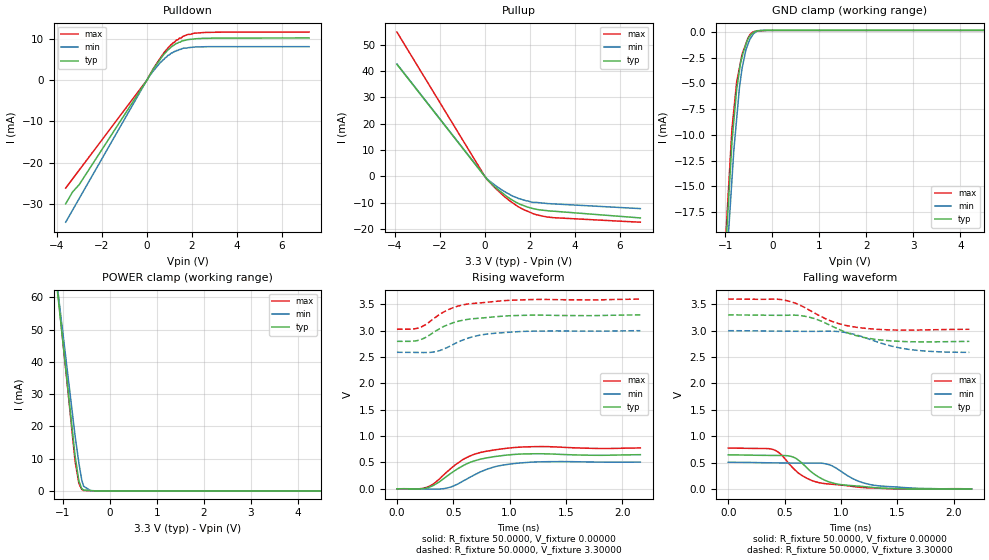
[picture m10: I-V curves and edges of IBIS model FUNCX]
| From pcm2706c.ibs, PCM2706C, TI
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[Model] FUNCX
Model_type I/O
Vinl  = 800.000mV
Vinh  = 2.00000V
Vref  = 0.00000V
Cref  = 2.00000pF
Vmeas = 1.65000V
C_comp  2.00000pF 2.00000pF 2.00000pF
| variable   typ   min   max
[Voltage Range]   3.30000V  3.00000V  3.60000V
[POWER Clamp Reference]  3.30000V  3.00000V  3.60000V
[Pullup Reference]   3.30000V  3.00000V  3.60000V
[Pulldown Reference]   0.00000V  0.00000V  0.00000V
[GND Clamp Reference]   0.00000V  0.00000V  0.00000V
[Temperature Range]   25   85   -25
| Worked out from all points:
|   slope of the pulldown table from 0 to 0.495 V, typ, clamps not added: 114 ohm
|   slope of the pullup table from 0 to 0.495 V, typ, clamps not added: 116 ohm
|   GND clamp passes 1 mA (typ) near -0.55 V on its own axis
|   POWER clamp passes 1 mA (typ) near -0.61 V on its own axis
|   rising waveform, R_fixture 50.0000, V_fixture 0.00000: 20-80 % time 296ps typ, 298ps min, 286ps max; typ from 0 V to 0.648 V
|   falling waveform, R_fixture 50.0000, V_fixture 0.00000: 20-80 % time 263ps typ, 275ps min, 265ps max; typ from 0.648 V to 0 V
|   falling waveform, R_fixture 50.0000, V_fixture 3.30000: 20-80 % time 347ps typ, 388ps min, 335ps max; typ from 3.3 V to 2.8 V
|   rising waveform, R_fixture 50.0000, V_fixture 3.30000: 20-80 % time 312ps typ, 307ps min, 303ps max; typ from 2.8 V to 3.3 V
[GND Clamp]
-3.3V     -202.3mA   -188.4mA   -204.3mA
-861.2mV  -10.72mA   -14.36mA   -9.41mA
-820.9mV  -8.663mA   -11.49mA   -7.586mA
-760.1mV  -5.554mA   -8.402mA   -4.835mA
-699.5mV  -3.669mA   -5.325mA   -3.426mA
-643.8mV  -2.39mA    -3.477mA   -2.13mA
-562.3mV  -1.186mA   -1.697mA   -1.114mA
-502mV    -524.1uA   -970uA     -443.3uA
-421mV    -152uA     -289.9uA   1.582uA
-310.9mV  131.6uA    135.8uA    112.4uA
-181.8mV  165.3uA    158.2uA    136.9uA
6.6V      176.1uA    158.9uA    160.8uA
[Pulldown]
-3.6V     -29.93mA   -34.38mA   -26.13mA
-3.3V     -27.11mA   -31.52mA   -23.96mA
-3V       -25.3mA    -28.66mA   -21.79mA
20.8mV    92.19uA    132.4uA    70.78uA
299.7mV   2.737mA    2.231mA    2.811mA
800.2mV   6.424mA    5.253mA    6.883mA
941.6mV   7.269mA    5.945mA    7.724mA
1.179V    8.327mA    6.76mA     9.042mA
1.442V    9.105mA    7.336mA    10.09mA
2.079V    9.887mA    7.918mA    11.27mA
3.499V    10.1mA     8.032mA    11.56mA
7.2V      10.15mA    8.034mA    11.56mA
[Pullup]
-3.9V     42.53mA    42.65mA    54.78mA
0V        -82.33uA   20.74uA    -14.22uA
179.3mV   -1.837mA   -1.58mA    -1.929mA
478.1mV   -4.227mA   -3.543mA   -4.596mA
1.039V    -8.041mA   -6.567mA   -8.869mA
1.459V    -10.16mA   -8.298mA   -11.43mA
1.79V     -11.41mA   -9.183mA   -12.89mA
2.257V    -12.47mA   -9.921mA   -14.51mA
2.778V    -13.05mA   -10.35mA   -15.46mA
6.9V      -15.8mA    -12.27mA   -17.43mA
[POWER Clamp]
-3.3V     358.5mA    330.7mA    375.2mA
-1.039V   51.39mA    53.61mA    51.84mA
-741.1mV  10.88mA    17.07mA    9.188mA
-660.1mV  3.071mA    8.621mA    2.296mA
-599.6mV  727.7uA    3.402mA    494.6uA
-559.1mV  265uA      1.442mA    152.2uA
-402.1mV  116.2uA    5.961uA    32.75uA
6.6V      0A         0A         0A
[Rising Waveform]
R_fixture = 50.0000
V_fixture = 0.00000
V_fixture_min = 0.00000
V_fixture_max = 0.00000
0s        0V         0V         0V
200ps     -1.778mV   -1.272mV   671.5uV
280ps     26.47mV    -4.28mV    41.9mV
440ps     234.3mV    13.08mV    315.2mV
580ps     431.4mV    138.7mV    548.5mV
680ps     525.6mV    256.3mV    651.2mV
800ps     587.8mV    372.9mV    715mV
940ps     631.5mV    450.1mV    760.2mV
1.2ns     664.2mV    506.4mV    799.1mV
2.16ns    647.7mV    506.2mV    775.6mV
[Falling Waveform]
R_fixture = 50.0000
V_fixture = 0.00000
V_fixture_min = 0.00000
V_fixture_max = 0.00000
0s        647.7mV    506.2mV    775.6mV
400ps     635.4mV    495mV      746.9mV
460ps     635mV      493.5mV    672.1mV
580ps     601.7mV    490.9mV    385.5mV
700ps     397.6mV    489.9mV    201.3mV
820ps     206.5mV    489.6mV    113.8mV
980ps     89.29mV    365.3mV    79.05mV
1.14ns    56.55mV    161.8mV    38.61mV
1.28ns    29.32mV    75.53mV    18.37mV
2.16ns    0V         0V         0V
[Falling Waveform]
R_fixture = 50.0000
V_fixture = 3.30000
V_fixture_min = 3.00000
V_fixture_max = 3.60000
0s        3.3V       3V         3.6V
460ps     3.292V     2.992V     3.592V
560ps     3.295V     2.99V      3.547V
680ps     3.274V     2.988V     3.439V
780ps     3.219V     2.988V     3.319V
920ps     3.087V     2.991V     3.178V
1.18ns    2.884V     2.894V     3.053V
1.4ns     2.815V     2.736V     3.019V
1.58ns    2.793V     2.654V     3.011V
2.14ns    2.798V     2.59V      3.027V
[Rising Waveform]
R_fixture = 50.0000
V_fixture = 3.30000
V_fixture_min = 3.00000
V_fixture_max = 3.60000
0s        2.798V     2.59V      3.027V
120ps     2.799V     2.589V     3.029V
200ps     2.823V     2.586V     3.057V
260ps     2.879V     2.586V     3.122V
340ps     2.989V     2.601V     3.25V
480ps     3.136V     2.718V     3.421V
640ps     3.218V     2.864V     3.509V
800ps     3.249V     2.937V     3.54V
1.12ns    3.291V     2.986V     3.586V
2.16ns    3.3V       3V         3.6V
[Ramp]
| variable typ   min   max
dV/dt_r   386.302m/420.508p  302.371m/472.835p  463.460m/391.970p
dV/dt_f   303.967m/426.304p  240.198m/473.539p  345.648m/394.914p
R_load  =  50.0000Ohms
